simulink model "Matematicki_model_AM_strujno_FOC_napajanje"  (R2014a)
settings: Solver=ode3  StartTime=0.0  StopTime=Tfinalno  FixedStep=Tsim  RelTol=1e-3
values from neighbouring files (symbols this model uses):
  A1 = [-1/Tr 0; 0 -1/Tr]    [Matematicki_model_AM_strujno_FOC_napajanje_parametri.m]
  A2 = [0 1; -1 0]    [Matematicki_model_AM_strujno_FOC_napajanje_parametri.m]
  A3 = [0 -1; 1 0]    [Matematicki_model_AM_strujno_FOC_napajanje_parametri.m]
  Am = [-Kfv*p/J -Kel*p/J; 1 0]    [Matematicki_model_AM_strujno_FOC_napajanje_parametri.m]
  B = [Lm/Tr 0; 0 Lm/Tr]    [Matematicki_model_AM_strujno_FOC_napajanje_parametri.m]
  Bm = [p/J -p/J; 0 0]    [Matematicki_model_AM_strujno_FOC_napajanje_parametri.m]
  Isd_ref = 2.0    (= 2)    [Matematicki_model_AM_strujno_FOC_napajanje_parametri.m]
  Isq_ref = 0.5    [Matematicki_model_AM_strujno_FOC_napajanje_parametri.m]
  Kp = 5000    [Matematicki_model_AM_strujno_FOC_napajanje_parametri.m]
  Lm = 0.422    [Matematicki_model_AM_strujno_FOC_napajanje_parametri.m]
  Lr = Lxr+Lm    (= 0.462)    [Matematicki_model_AM_strujno_FOC_napajanje_parametri.m]
  Lsigma = Ls*sigm    (= 0.0765367965368)    [Matematicki_model_AM_strujno_FOC_napajanje_parametri.m]
  p = 2    [Matematicki_model_AM_strujno_FOC_napajanje_parametri.m]
  Rs = 10.0    (= 10)    [Matematicki_model_AM_strujno_FOC_napajanje_parametri.m]
  t_flux = 1.0    (= 1)    [Matematicki_model_AM_strujno_FOC_napajanje_parametri.m]
  t_me = 3.0    (= 3)    [Matematicki_model_AM_strujno_FOC_napajanje_parametri.m]
  Tn = 1000*Tr    (= 73.3333333333)    [Matematicki_model_AM_strujno_FOC_napajanje_parametri.m]
  Tr_FOC = Tr    (= 0.0733333333333)    [Matematicki_model_AM_strujno_FOC_napajanje_parametri.m]
  TROUGAO_ZVEZDA = 0    [Matematicki_model_AM_strujno_FOC_napajanje_parametri.m]
  Tsim = Tpwm/16    (= 3.125e-06)    [Matematicki_model_AM_strujno_FOC_napajanje_parametri.m]
libraries: simulink x1

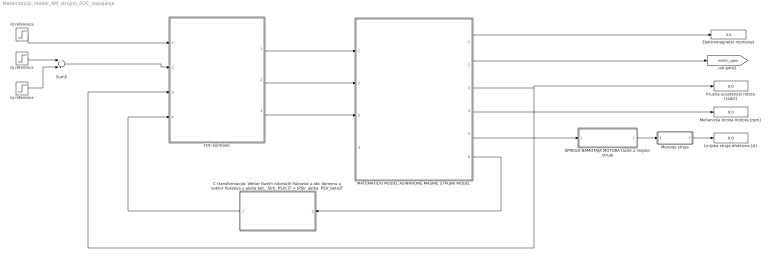
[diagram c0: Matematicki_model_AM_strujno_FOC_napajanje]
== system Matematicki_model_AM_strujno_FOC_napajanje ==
  " Iq referenca " : Step  Time=t_me+0.5  After=Isq_ref  SampleTime=Tsim
  C transformacija: Vektor faznih rotorskih flukseva u abc domenu u vektor flukseva u alpha beta referentnom sistemu - [PSIra  PSIrb  PSIrc]T = [PSIr_alpha  PSIr_beta]T : Subsystem
  Elektromagnetni momenat : Display
  FOC kontroler : Subsystem
  Id referenca : Step  Time=t_flux  After=Isd_ref  SampleTime=Tsim
  Iq referenca : Step  Time=t_me  After=Isq_ref  SampleTime=Tsim
  Kruzna ucestanost rotora [rad/s] : Display
  Linijska struja efektivno [A] : Display
  MATEMATICKI MODEL ASINHRONE MASINE STRUJNI MODEL : Subsystem
  Mehanicka brzina motora [rpm] : Display
  Merenje struje : Subsystem
  SPREGA NAMOTAJA MOTORA fazne u linijske struje : Subsystem
  Sum5 : Sum  Inputs=+-  SampleTime=Tsim
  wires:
  Merenje struje/1(Is_eff) -> Linijska struja efektivno [A]/1
  MATEMATICKI MODEL ASINHRONE MASINE STRUJNI MODEL/5(" Is_abc ") -> SPREGA NAMOTAJA MOTORA fazne u linijske struje/1(Is_abc fazno)
  MATEMATICKI MODEL ASINHRONE MASINE STRUJNI MODEL/4(Brzina meh [o/min]) -> Mehanicka brzina motora [rpm]/1
  MATEMATICKI MODEL ASINHRONE MASINE STRUJNI MODEL/1(M_el) -> Elektromagnetni momenat/1
  MATEMATICKI MODEL ASINHRONE MASINE STRUJNI MODEL/2(ugao rot_el) -> [motor_ugao]
  Iq referenca/1 -> Sum5/1
  " Iq referenca "/1 -> Sum5/2
  SPREGA NAMOTAJA MOTORA fazne u linijske struje/1("Is_abc invertor ") -> Merenje struje/1(Is_abc)
  MATEMATICKI MODEL ASINHRONE MASINE STRUJNI MODEL/6(PSIr_abc) -> C transformacija: Vektor faznih rotorskih flukseva u abc domenu u vektor flukseva u alpha beta referentnom sistemu - [PSIra  PSIrb  PSIrc]T = [PSIr_alpha  PSIr_beta]T/1(PSIr_abc)
  MATEMATICKI MODEL ASINHRONE MASINE STRUJNI MODEL/3(wr_el) -> FOC kontroler/3(w el), Kruzna ucestanost rotora [rad/s]/1
  Id referenca/1 -> FOC kontroler/1(Isd)
  Sum5/1 -> FOC kontroler/2(Isq)
  C transformacija: Vektor faznih rotorskih flukseva u abc domenu u vektor flukseva u alpha beta referentnom sistemu - [PSIra  PSIrb  PSIrc]T = [PSIr_alpha  PSIr_beta]T/1(PSIr_alphabeta) -> FOC kontroler/4(PSIr)
  FOC kontroler/1(Is_abc) -> MATEMATICKI MODEL ASINHRONE MASINE STRUJNI MODEL/1(Is_abc)
  FOC kontroler/2(wdq) -> MATEMATICKI MODEL ASINHRONE MASINE STRUJNI MODEL/2(W_dq)
  FOC kontroler/3(ugao_dq) -> MATEMATICKI MODEL ASINHRONE MASINE STRUJNI MODEL/3(ugao_dq)

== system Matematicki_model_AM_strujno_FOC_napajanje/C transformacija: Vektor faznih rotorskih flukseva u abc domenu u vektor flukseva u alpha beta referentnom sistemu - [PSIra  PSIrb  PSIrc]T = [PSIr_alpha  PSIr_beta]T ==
  PSIr_abc : Inport
  Isb : Fcn  Expr=2/3*(0*u[1]+sqrt(3)/2*u[2]-sqrt(3)/2*u[3])  SampleTime=Tsim
  Mux1 : Mux  Inputs=2
  PSI_alpha : Fcn  Expr=2/3*(1*u[1]-1/2*u[2]-1/2*u[3])  SampleTime=Tsim
  PSIr_alphabeta : Outport
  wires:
  PSIr_abc/1 -> Isb/1, PSI_alpha/1
  PSI_alpha/1 -> Mux1/1
  Isb/1 -> Mux1/2
  Mux1/1 -> PSIr_alphabeta/1

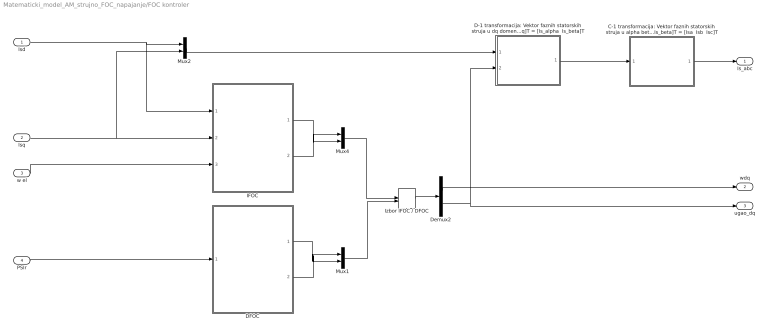
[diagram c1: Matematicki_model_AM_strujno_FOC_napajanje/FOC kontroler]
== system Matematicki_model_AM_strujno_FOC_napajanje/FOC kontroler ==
  Isd : Inport
  Isq : Inport  Port=2
  w el : Inport  Port=3
  PSIr : Inport  Port=4
  C-1 transformacija: Vektor faznih statorskih struja u alpha beta domenu u vektor struja u abc referentnom sistemu - [Is_alpha  Is_beta]T = [Isa  Isb  Isc]T : Subsystem
  D-1 transformacija: Vektor faznih statorskih struja u dq domenu u vektor struja u alpha beta referentnom sistemu - [Isd  Isq]T = [Is_alpha  Is_beta]T : Subsystem
  DFOC : Subsystem
  Demux2 : Demux  Outputs=2
  IFOC : Subsystem
  Izbor IFOC / DFOC : ManualSwitch
  Mux1 : Mux  Inputs=2
  Mux2 : Mux  Inputs=2
  Mux4 : Mux  Inputs=2
  Is_abc : Outport
  wdq : Outport  Port=2
  ugao_dq : Outport  Port=3
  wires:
  Mux2/1 -> D-1 transformacija: Vektor faznih statorskih struja u dq domenu u vektor struja u alpha beta referentnom sistemu - [Isd  Isq]T = [Is_alpha  Is_beta]T/1(Is_dq)
  Isq/1 -> Mux2/2, IFOC/2(Isq)
  Isd/1 -> IFOC/1(Isd), Mux2/1
  PSIr/1 -> DFOC/1(PSIr)
  D-1 transformacija: Vektor faznih statorskih struja u dq domenu u vektor struja u alpha beta referentnom sistemu - [Isd  Isq]T = [Is_alpha  Is_beta]T/1(Is_alpha_beta) -> C-1 transformacija: Vektor faznih statorskih struja u alpha beta domenu u vektor struja u abc referentnom sistemu - [Is_alpha  Is_beta]T = [Isa  Isb  Isc]T/1(Is_alphabeta)
  C-1 transformacija: Vektor faznih statorskih struja u alpha beta domenu u vektor struja u abc referentnom sistemu - [Is_alpha  Is_beta]T = [Isa  Isb  Isc]T/1(Is_abc) -> Is_abc/1
  Izbor IFOC / DFOC/1 -> Demux2/1
  IFOC/2(ugao_IFOC) -> Mux4/2
  Demux2/2 -> D-1 transformacija: Vektor faznih statorskih struja u dq domenu u vektor struja u alpha beta referentnom sistemu - [Isd  Isq]T = [Is_alpha  Is_beta]T/2(ugao_dq), ugao_dq/1
  IFOC/1(brzina_IFOC) -> Mux4/1
  DFOC/2(ugao_DFOC) -> Mux1/2
  Mux4/1 -> Izbor IFOC / DFOC/1
  DFOC/1(brzina_DFOC) -> Mux1/1
  Mux1/1 -> Izbor IFOC / DFOC/2
  Demux2/1 -> wdq/1
  w el/1 -> IFOC/3(w el)

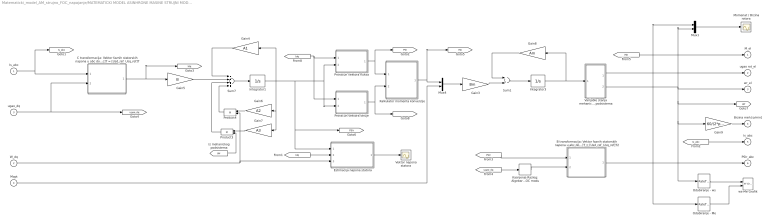
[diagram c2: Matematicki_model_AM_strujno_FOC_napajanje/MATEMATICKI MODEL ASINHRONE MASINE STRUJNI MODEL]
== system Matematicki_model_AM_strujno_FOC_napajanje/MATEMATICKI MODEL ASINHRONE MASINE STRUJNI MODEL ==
  Is_abc : Inport
  W_dq : Inport  Port=2
  ugao_dq : Inport  Port=3
  Mopt : Inport  Port=4
  B transformacija: Vektor faznih statorskih napona u abc domenu u vektor napona u dq referentnom sistemu - [Usa  Usb Usc]T = [Usd_ref  Usq_ref]T2 : Subsystem
  C transformacija: Vektor faznih statorskih napona u abc domenu u vektor napona u dq referentnom sistemu - [Usa  Usb Usc]T = [Usd_ref  Usq_ref]T : Subsystem
  Estimacija napona statora : Subsystem
  Gain3 : Gain  Gain=Bm  Multiplication=Matrix(K*u) (u vector)  SampleTime=Tsim
  Gain4 : Gain  Gain=A1  Multiplication=Matrix(K*u) (u vector)  SampleTime=Tsim
  Gain5 : Gain  Gain=B  Multiplication=Matrix(K*u) (u vector)  SampleTime=Tsim
  Gain6 : Gain  Gain=A2  Multiplication=Matrix(K*u) (u vector)  SampleTime=Tsim
  Gain7 : Gain  Gain=A3  Multiplication=Matrix(K*u) (u vector)  SampleTime=Tsim
  Gain8 : Gain  Gain=Am  Multiplication=Matrix(K*u) (u vector)  SampleTime=Tsim
  Gain9 : Gain  Gain=60/(2*pi()*p)  SampleTime=Tsim
  Integrator1 : Integrator  InitialCondition=[0,0]
  Integrator3 : Integrator  InitialCondition=[0,0]
  Kalkulator momenta konverzije : Subsystem
  Kasnjenje Razlog: Algebarska petlja u DFOC modu : Delay  DelayLength=1  SampleTime=Tsim
  Momenat / Brzina rotora : Scope
  Mux1 : Mux  Inputs=2
  Mux4 : Mux  Inputs=2
  Odabiranje - Me : RateTransition  OutPortSampleTime=100*Tsim
  Odabiranje - ws : RateTransition  OutPortSampleTime=100*Tsim
  Product3 : Product  SampleTime=Tsim
  Product4 : Product  SampleTime=Tsim
  Proracun vektora fluksa : Subsystem
  Proracun vektora struje : Subsystem
  Sum1 : Sum  SampleTime=Tsim
  Sum7 : Sum  Inputs=++++  SampleTime=Tsim
  Varijable stanja mehanickog podsistema : Subsystem
  Vektor napona statora : Scope
  ws-Me Grafik : simulink/Sinks/XY Graph  xmin=-400  xmax=400  ymin=-5  ymax=5  st=100*Tsim
  M_el : Outport  InitialOutput=0
  ugao rot_el : Outport  Port=2  InitialOutput=0
  wr_el : Outport  Port=3  InitialOutput=0
  Brzina meh [o/min] : Outport  Port=4  InitialOutput=0
  " Is_abc " : Outport  Port=5  InitialOutput=0
  PSIr_abc : Outport  Port=6  InitialOutput=0
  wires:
  Odabiranje - Me/1 -> ws-Me Grafik/2
  Odabiranje - ws/1 -> ws-Me Grafik/1
  Mux1/1 -> Momenat / Brzina rotora/1
  [Is_abc] -> " Is_abc "/1
  Integrator3/1 -> Gain8/1, Varijable stanja mehanickog podsistema/1(X2)
  Gain8/1 -> Sum1/1
  Sum1/1 -> Integrator3/1
  Gain3/1 -> Sum1/2
  Mux4/1 -> Gain3/1
  Gain9/1 -> Brzina meh [o/min]/1
  Varijable stanja mehanickog podsistema/2(w) -> Mux1/2, Odabiranje - ws/1, Gain9/1, [Wr], wr_el/1
  Varijable stanja mehanickog podsistema/1(theta) -> ugao rot_el/1
  [Me] -> Mux1/1, Odabiranje - Me/1, M_el/1
  Mopt/1 -> Mux4/2
  Kalkulator momenta konverzije/1(Me) -> Mux4/1, [Me]
  Proracun vektora struje/1(I) -> Kalkulator momenta konverzije/2(I), [I]
  Proracun vektora fluksa/1(PSI) -> Kalkulator momenta konverzije/1(PSI), [PSI]
  Product4/1 -> Sum7/4
  W_dq/1 -> Product4/2, Estimacija napona statora/3(wdq)
  Gain5/1 -> Sum7/2
  Gain4/1 -> Sum7/1
  Sum7/1 -> Integrator1/1
  Gain6/1 -> Product4/1
  Gain7/1 -> Product3/1
  Product3/1 -> Sum7/3
  [Wr] -> Product3/2
  [Idq] -> Proracun vektora fluksa/1(Is), Proracun vektora struje/1(Is)
  Estimacija napona statora/1(Vs) -> Vektor napona statora/1
  [Idq] -> Estimacija napona statora/2(Is)
  Integrator1/1 -> Gain6/1, Gain7/1, [PSIr], Estimacija napona statora/1(PSIr), Proracun vektora struje/2(PSIr), Proracun vektora fluksa/2(PSIr), Gain4/1
  Is_abc/1 -> [Is_abc], C transformacija: Vektor faznih statorskih napona u abc domenu u vektor napona u dq referentnom sistemu - [Usa  Usb Usc]T = [Usd_ref  Usq_ref]T/1(Is_abc)
  C transformacija: Vektor faznih statorskih napona u abc domenu u vektor napona u dq referentnom sistemu - [Usa  Usb Usc]T = [Usd_ref  Usq_ref]T/1(Is_dq) -> [Idq], Gain5/1
  B transformacija: Vektor faznih statorskih napona u abc domenu u vektor napona u dq referentnom sistemu - [Usa  Usb Usc]T = [Usd_ref  Usq_ref]T2/1(PSIr_abc) -> PSIr_abc/1
  [PSIr] -> B transformacija: Vektor faznih statorskih napona u abc domenu u vektor napona u dq referentnom sistemu - [Usa  Usb Usc]T = [Usd_ref  Usq_ref]T2/1(PSIr_dq)
  ugao_dq/1 -> [ugao_dq], C transformacija: Vektor faznih statorskih napona u abc domenu u vektor napona u dq referentnom sistemu - [Usa  Usb Usc]T = [Usd_ref  Usq_ref]T/2(ugao_dq)
  [ugao_dq] -> Kasnjenje Razlog: Algebarska petlja u DFOC modu/1
  Kasnjenje Razlog: Algebarska petlja u DFOC modu/1 -> B transformacija: Vektor faznih statorskih napona u abc domenu u vektor napona u dq referentnom sistemu - [Usa  Usb Usc]T = [Usd_ref  Usq_ref]T2/2(ugao_dq)

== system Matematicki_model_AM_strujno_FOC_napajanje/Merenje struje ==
  Is_abc : Inport
  Is_alfa : Fcn  Expr=(2/3)*(u[1]-(u[2]+u[3])/2)  SampleTime=Tsim
  Is_amplituda : Fcn  Expr=sqrt(u[1]^2+u[2]^2)/sqrt(2)  SampleTime=Tsim
  Is_beta : Fcn  Expr=(u[2]-u[3])/sqrt(3)  SampleTime=Tsim
  Mux : Mux  Inputs=2
  Is_eff : Outport
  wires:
  Is_abc/1 -> Is_beta/1, Is_alfa/1
  Is_alfa/1 -> Mux/1
  Is_beta/1 -> Mux/2
  Mux/1 -> Is_amplituda/1
  Is_amplituda/1 -> Is_eff/1

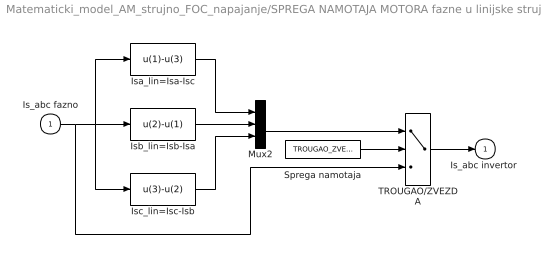
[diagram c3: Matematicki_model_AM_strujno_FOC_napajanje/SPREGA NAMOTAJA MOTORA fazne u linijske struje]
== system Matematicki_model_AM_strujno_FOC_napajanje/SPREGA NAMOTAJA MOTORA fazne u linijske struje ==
  Is_abc fazno : Inport
  Isa_lin=Isa-Isc : Fcn  Expr=u(1)-u(3)  SampleTime=Tsim
  Isb_lin=Isb-Isa : Fcn  Expr=u(2)-u(1)  SampleTime=Tsim
  Isc_lin=Isc-Isb : Fcn  Expr=u(3)-u(2)  SampleTime=Tsim
  Mux2 : Mux  Inputs=3
  Sprega namotaja : Constant  Value=TROUGAO_ZVEZDA
  TROUGAO/ZVEZDA : Switch  Threshold=0.1  SampleTime=Tsim
  "Is_abc invertor " : Outport  InitialOutput=0
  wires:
  Sprega namotaja/1 -> TROUGAO/ZVEZDA/2
  Mux2/1 -> TROUGAO/ZVEZDA/1
  TROUGAO/ZVEZDA/1 -> "Is_abc invertor "/1
  Is_abc fazno/1 -> TROUGAO/ZVEZDA/3, Isa_lin=Isa-Isc/1, Isb_lin=Isb-Isa/1, Isc_lin=Isc-Isb/1
  Isa_lin=Isa-Isc/1 -> Mux2/1
  Isb_lin=Isb-Isa/1 -> Mux2/2
  Isc_lin=Isc-Isb/1 -> Mux2/3

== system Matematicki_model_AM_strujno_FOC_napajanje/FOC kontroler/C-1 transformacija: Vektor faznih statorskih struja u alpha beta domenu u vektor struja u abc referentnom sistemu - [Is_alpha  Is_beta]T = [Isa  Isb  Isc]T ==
  Is_alphabeta : Inport
  Isa : Fcn  Expr=(1*u[1]-0*u[2])  SampleTime=Tsim
  Isb : Fcn  Expr=(-1/2*u[1]+sqrt(3)/2*u[2])  SampleTime=Tsim
  Isc : Fcn  Expr=(-1/2*u[1]-sqrt(3)/2*u[2])  SampleTime=Tsim
  Mux1 : Mux  Inputs=3
  Is_abc : Outport
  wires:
  Isc/1 -> Mux1/3
  Is_alphabeta/1 -> Isa/1, Isb/1, Isc/1
  Isa/1 -> Mux1/1
  Isb/1 -> Mux1/2
  Mux1/1 -> Is_abc/1

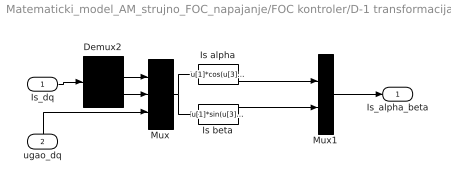
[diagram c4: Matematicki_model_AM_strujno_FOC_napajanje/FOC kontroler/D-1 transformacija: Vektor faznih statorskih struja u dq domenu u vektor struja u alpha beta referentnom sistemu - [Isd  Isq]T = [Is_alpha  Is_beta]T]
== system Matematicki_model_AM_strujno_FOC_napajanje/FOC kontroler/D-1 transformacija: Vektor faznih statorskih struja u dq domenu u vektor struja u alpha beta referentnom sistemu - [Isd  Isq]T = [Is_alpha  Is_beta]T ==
  Is_dq : Inport
  ugao_dq : Inport  Port=2
  Demux2 : Demux  Outputs=2
  Is alpha : Fcn  Expr=u[1]*cos(u[3])-u[2]*sin(u[3])  SampleTime=Tsim
  Is beta : Fcn  Expr=u[1]*sin(u[3])+u[2]*cos(u[3])  SampleTime=Tsim
  Mux : Mux  Inputs=3
  Mux1 : Mux  Inputs=2
  Is_alpha_beta : Outport
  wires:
  Is alpha/1 -> Mux1/1
  Is beta/1 -> Mux1/2
  Mux/1 -> Is beta/1, Is alpha/1
  Demux2/2 -> Mux/2
  Demux2/1 -> Mux/1
  ugao_dq/1 -> Mux/3
  Is_dq/1 -> Demux2/1
  Mux1/1 -> Is_alpha_beta/1

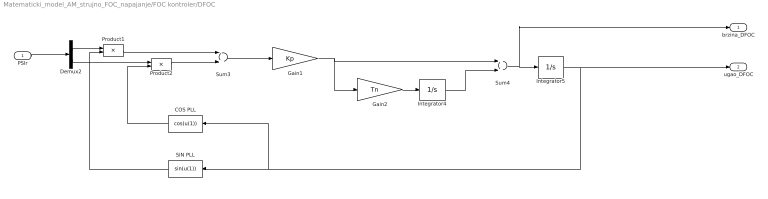
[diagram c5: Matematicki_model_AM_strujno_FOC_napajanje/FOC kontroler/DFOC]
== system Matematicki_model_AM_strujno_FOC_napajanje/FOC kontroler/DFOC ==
  PSIr : Inport
  COS PLL : Fcn  Expr=cos(u(1))  SampleTime=Tsim
  Demux2 : Demux  Outputs=2
  Gain1 : Gain  Gain=Kp  SampleTime=Tsim
  Gain2 : Gain  Gain=Tn  SampleTime=Tsim
  Integrator4 : Integrator  InitialCondition=[0]
  Integrator5 : Integrator  InitialCondition=[0]
  Product1 : Product  SampleTime=Tsim
  Product2 : Product  SampleTime=Tsim
  SIN PLL : Fcn  Expr=sin(u(1))  SampleTime=Tsim
  Sum3 : Sum  Inputs=-+  SampleTime=Tsim
  Sum4 : Sum  SampleTime=Tsim
  brzina_DFOC : Outport
  ugao_DFOC : Outport  Port=2
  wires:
  SIN PLL/1 -> Product1/2
  Product2/1 -> Sum3/2
  Demux2/2 -> Product2/1
  Gain2/1 -> Integrator4/1
  COS PLL/1 -> Product2/2
  Integrator5/1 -> ugao_DFOC/1, COS PLL/1, SIN PLL/1
  Demux2/1 -> Product1/1
  Product1/1 -> Sum3/1
  Gain1/1 -> Gain2/1, Sum4/1
  Sum3/1 -> Gain1/1
  PSIr/1 -> Demux2/1
  Sum4/1 -> brzina_DFOC/1, Integrator5/1
  Integrator4/1 -> Sum4/2

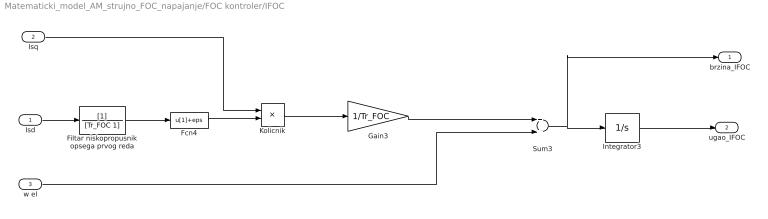
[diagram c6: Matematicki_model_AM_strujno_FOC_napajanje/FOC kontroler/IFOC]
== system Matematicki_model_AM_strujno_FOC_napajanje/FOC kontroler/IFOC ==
  Isd : Inport
  Isq : Inport  Port=2
  w el : Inport  Port=3
  Fcn4 : Fcn  Expr=u[1]+eps  SampleTime=Tsim
  Filtar niskopropusnik opsega prvog reda : TransferFcn  Denominator=[Tr_FOC 1]
  Gain3 : Gain  Gain=1/Tr_FOC  SampleTime=Tsim
  Integrator3 : Integrator  InitialCondition=[0]
  Kolicnik : Product  Inputs=*/  SampleTime=Tsim
  Sum3 : Sum  SampleTime=Tsim
  brzina_IFOC : Outport
  ugao_IFOC : Outport  Port=2
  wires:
  w el/1 -> Sum3/2
  Integrator3/1 -> ugao_IFOC/1
  Isq/1 -> Kolicnik/1
  Sum3/1 -> brzina_IFOC/1, Integrator3/1
  Kolicnik/1 -> Gain3/1
  Gain3/1 -> Sum3/1
  Filtar niskopropusnik opsega prvog reda/1 -> Fcn4/1
  Isd/1 -> Filtar niskopropusnik opsega prvog reda/1
  Fcn4/1 -> Kolicnik/2

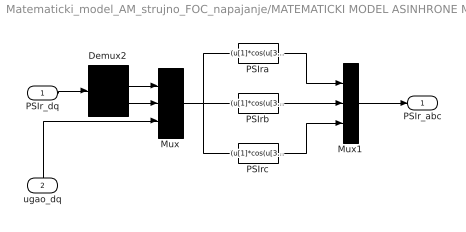
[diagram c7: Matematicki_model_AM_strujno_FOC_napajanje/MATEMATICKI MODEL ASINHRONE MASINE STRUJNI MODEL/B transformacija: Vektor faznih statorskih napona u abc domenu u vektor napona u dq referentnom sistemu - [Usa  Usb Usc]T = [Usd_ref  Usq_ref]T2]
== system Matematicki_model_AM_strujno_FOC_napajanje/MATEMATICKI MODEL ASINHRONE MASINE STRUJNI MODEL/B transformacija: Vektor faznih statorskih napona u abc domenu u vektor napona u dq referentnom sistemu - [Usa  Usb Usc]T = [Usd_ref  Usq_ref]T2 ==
  PSIr_dq : Inport
  ugao_dq : Inport  Port=2
  Demux2 : Demux  Outputs=2
  Mux : Mux  Inputs=3
  Mux1 : Mux  Inputs=3
  PSIra : Fcn  Expr=(u[1]*cos(u[3])-u[2]*sin(u[3]))  SampleTime=Tsim
  PSIrb : Fcn  Expr=(u[1]*cos(u[3]-2*pi/3)-u[2]*sin(u[3]-2*pi/3))  SampleTime=Tsim
  PSIrc : Fcn  Expr=(u[1]*cos(u[3]+2*pi/3)-u[2]*sin(u[3]+2*pi/3))  SampleTime=Tsim
  PSIr_abc : Outport
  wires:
  Mux1/1 -> PSIr_abc/1
  PSIr_dq/1 -> Demux2/1
  Demux2/1 -> Mux/1
  ugao_dq/1 -> Mux/3
  Demux2/2 -> Mux/2
  Mux/1 -> PSIrc/1, PSIra/1, PSIrb/1
  PSIrb/1 -> Mux1/2
  PSIra/1 -> Mux1/1
  PSIrc/1 -> Mux1/3

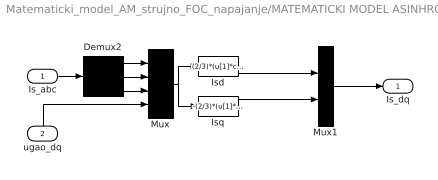
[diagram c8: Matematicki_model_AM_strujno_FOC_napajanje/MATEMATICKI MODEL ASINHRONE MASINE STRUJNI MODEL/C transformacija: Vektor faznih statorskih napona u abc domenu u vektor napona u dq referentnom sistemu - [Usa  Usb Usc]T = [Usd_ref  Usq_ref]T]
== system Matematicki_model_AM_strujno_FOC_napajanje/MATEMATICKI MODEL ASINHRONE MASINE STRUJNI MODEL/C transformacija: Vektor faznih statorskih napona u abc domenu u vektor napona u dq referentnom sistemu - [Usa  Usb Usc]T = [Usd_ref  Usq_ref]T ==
  Is_abc : Inport
  ugao_dq : Inport  Port=2
  Demux2 : Demux  Outputs=3
  Isd : Fcn  Expr=(2/3)*(u[1]*cos(u[4])+u[2]*cos(u[4]-2*pi/3)+u[3]*cos(u[4]-4*pi/3))  SampleTime=Tsim
  Isq : Fcn  Expr=-(2/3)*(u[1]*sin(u[4])+u[2]*sin(u[4]-2*pi/3)+u[3]*sin(u[4]-4*pi/3))  SampleTime=Tsim
  Mux : Mux
  Mux1 : Mux  Inputs=2
  Is_dq : Outport
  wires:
  Mux1/1 -> Is_dq/1
  Is_abc/1 -> Demux2/1
  ugao_dq/1 -> Mux/4
  Demux2/1 -> Mux/1
  Demux2/3 -> Mux/3
  Demux2/2 -> Mux/2
  Mux/1 -> Isd/1, Isq/1
  Isq/1 -> Mux1/2
  Isd/1 -> Mux1/1

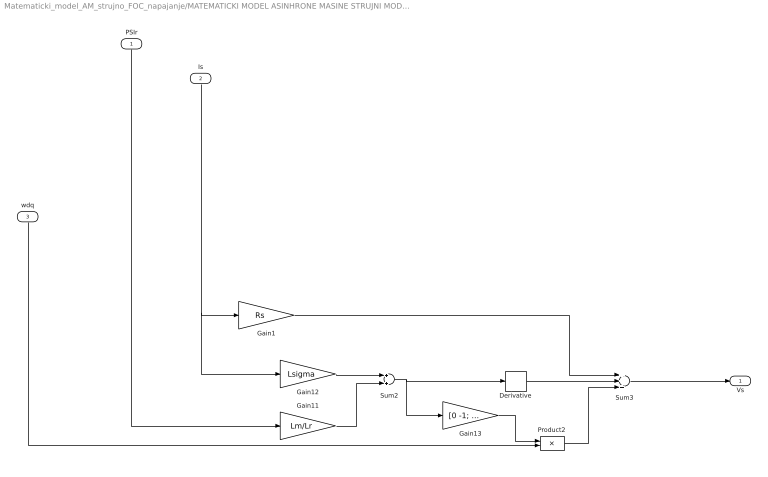
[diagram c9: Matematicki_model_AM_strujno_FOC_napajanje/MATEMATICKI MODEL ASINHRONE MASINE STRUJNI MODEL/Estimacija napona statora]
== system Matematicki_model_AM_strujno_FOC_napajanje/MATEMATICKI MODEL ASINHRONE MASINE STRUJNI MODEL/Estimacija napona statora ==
  PSIr : Inport
  Is : Inport  Port=2
  wdq : Inport  Port=3
  Derivative : Derivative
  Gain1 : Gain  Gain=Rs  SampleTime=Tsim
  Gain11 : Gain  Gain=Lm/Lr  SampleTime=Tsim
  Gain12 : Gain  Gain=Lsigma  SampleTime=Tsim
  Gain13 : Gain  Gain=[0 -1; 1 0]  Multiplication=Matrix(K*u) (u vector)  SampleTime=Tsim
  Product2 : Product  SampleTime=Tsim
  Sum2 : Sum  SampleTime=Tsim
  Sum3 : Sum  Inputs=+++  SampleTime=Tsim
  Vs : Outport
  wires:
  Gain11/1 -> Sum2/2
  Gain12/1 -> Sum2/1
  Sum2/1 -> Gain13/1, Derivative/1
  Product2/1 -> Sum3/3
  Sum3/1 -> Vs/1
  Gain1/1 -> Sum3/1
  Derivative/1 -> Sum3/2
  Gain13/1 -> Product2/1
  wdq/1 -> Product2/2
  PSIr/1 -> Gain11/1
  Is/1 -> Gain12/1, Gain1/1

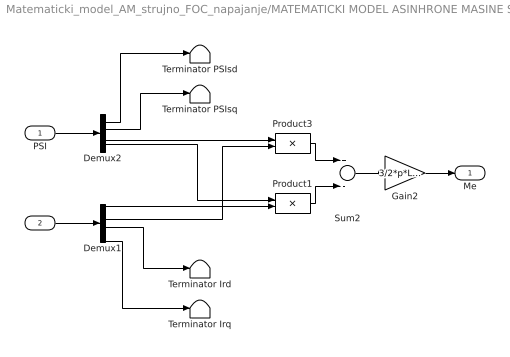
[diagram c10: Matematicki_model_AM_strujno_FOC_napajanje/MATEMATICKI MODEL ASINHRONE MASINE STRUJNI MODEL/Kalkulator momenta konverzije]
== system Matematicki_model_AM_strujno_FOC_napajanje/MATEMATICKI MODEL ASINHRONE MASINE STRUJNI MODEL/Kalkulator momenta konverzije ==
  PSI : Inport
  I : Inport  Port=2
  Demux1 : Demux
  Demux2 : Demux
  Gain2 : Gain  Gain=3/2*p*Lm/Lr  SampleTime=Tsim
  Product1 : Product  SampleTime=Tsim
  Product3 : Product  SampleTime=Tsim
  Sum2 : Sum  Inputs=+-  SampleTime=Tsim
  Terminator Ird : Terminator
  Terminator Irq : Terminator
  Terminator PSIsd : Terminator
  Terminator PSIsq : Terminator
  Me : Outport
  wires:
  Demux1/4 -> Terminator Irq/1
  Demux1/3 -> Terminator Ird/1
  Sum2/1 -> Gain2/1
  Gain2/1 -> Me/1
  Product1/1 -> Sum2/2
  Product3/1 -> Sum2/1
  Demux2/3 -> Product3/1
  Demux2/4 -> Product1/1
  I/1 -> Demux1/1
  Demux1/2 -> Product3/2
  Demux1/1 -> Product1/2
  Demux2/2 -> Terminator PSIsq/1
  Demux2/1 -> Terminator PSIsd/1
  PSI/1 -> Demux2/1

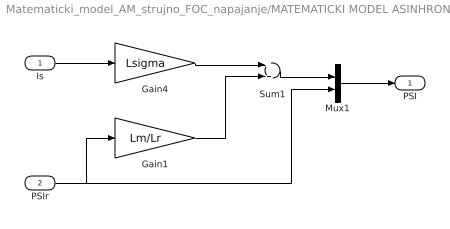
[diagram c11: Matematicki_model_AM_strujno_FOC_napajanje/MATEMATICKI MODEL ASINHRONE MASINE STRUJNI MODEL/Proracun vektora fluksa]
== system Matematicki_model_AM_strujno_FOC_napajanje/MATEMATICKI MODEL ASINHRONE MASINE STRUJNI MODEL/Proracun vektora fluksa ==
  Is : Inport
  PSIr : Inport  Port=2
  Gain1 : Gain  Gain=Lm/Lr  SampleTime=Tsim
  Gain4 : Gain  Gain=Lsigma  SampleTime=Tsim
  Mux1 : Mux  Inputs=2
  Sum1 : Sum  SampleTime=Tsim
  PSI : Outport
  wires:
  Sum1/1 -> Mux1/1
  Gain4/1 -> Sum1/1
  Gain1/1 -> Sum1/2
  PSIr/1 -> Mux1/2, Gain1/1
  Mux1/1 -> PSI/1
  Is/1 -> Gain4/1

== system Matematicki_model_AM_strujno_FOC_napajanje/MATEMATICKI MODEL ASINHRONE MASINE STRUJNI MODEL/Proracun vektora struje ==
  Is : Inport
  PSIr : Inport  Port=2
  Gain1 : Gain  Gain=Lm/Lr  SampleTime=Tsim
  Gain4 : Gain  Gain=1/Lr  SampleTime=Tsim
  Mux1 : Mux  Inputs=2
  Sum1 : Sum  Inputs=-+  SampleTime=Tsim
  I : Outport
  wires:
  Sum1/1 -> Mux1/2
  Gain4/1 -> Sum1/2
  Gain1/1 -> Sum1/1
  PSIr/1 -> Gain4/1
  Mux1/1 -> I/1
  Is/1 -> Mux1/1, Gain1/1

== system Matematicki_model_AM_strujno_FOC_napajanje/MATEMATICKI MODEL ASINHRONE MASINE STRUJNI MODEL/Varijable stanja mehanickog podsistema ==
  X2 : Inport
  Demux2 : Demux  Outputs=2
  theta : Outport
  w : Outport  Port=2
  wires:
  Demux2/1 -> w/1
  Demux2/2 -> theta/1
  X2/1 -> Demux2/1
